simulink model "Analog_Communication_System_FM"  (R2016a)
settings: Solver=ode3  StartTime=0.0  StopTime=6  FixedStep=1/5000000  RelTol=1e-3
libraries: dsparch4 x12, commsynccomp2 x8, simulink x8, commchan3 x2

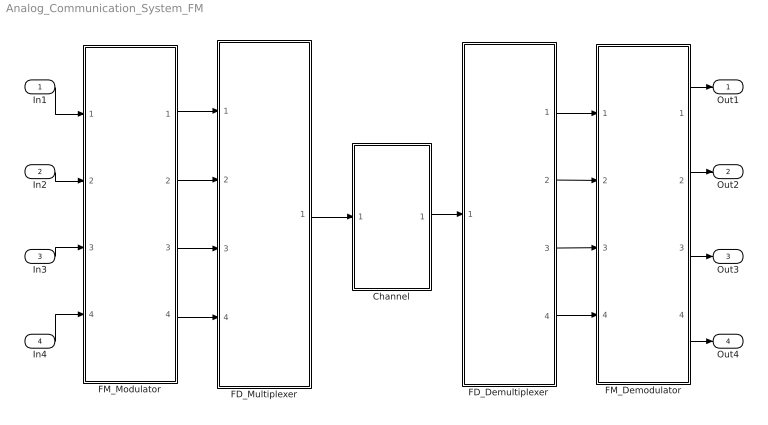
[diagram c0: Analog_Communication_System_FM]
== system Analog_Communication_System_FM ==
  In1 : Inport
  In2 : Inport  Port=2
  In3 : Inport  Port=3
  In4 : Inport  Port=4
  Channel : Subsystem
  FD_Demultiplexer : Subsystem
  FD_Multiplexer : Subsystem
  FM_Demodulator : Subsystem
  FM_Modulator : Subsystem
  Out1 : Outport
  Out2 : Outport  Port=2
  Out3 : Outport  Port=3
  Out4 : Outport  Port=4
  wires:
  In1/1 -> FM_Modulator/1(In1)
  In2/1 -> FM_Modulator/2(In2)
  In3/1 -> FM_Modulator/3(In3)
  In4/1 -> FM_Modulator/4(In4)
  FM_Modulator/1(Out1) -> FD_Multiplexer/1(In1)
  FM_Modulator/2(Out2) -> FD_Multiplexer/2(In2)
  FM_Modulator/3(Out3) -> FD_Multiplexer/3(In3)
  FM_Modulator/4(Out4) -> FD_Multiplexer/4(In4)
  FD_Multiplexer/1(Out) -> Channel/1(In1)
  Channel/1(Out1) -> FD_Demultiplexer/1(Input)
  FD_Demultiplexer/1(Out1) -> FM_Demodulator/1(In1)
  FD_Demultiplexer/2(Out2) -> FM_Demodulator/2(In2)
  FD_Demultiplexer/3(Out3) -> FM_Demodulator/3(In3)
  FD_Demultiplexer/4(Out4) -> FM_Demodulator/4(In4)
  FM_Demodulator/1(Out1) -> Out1/1
  FM_Demodulator/2(Out2) -> Out2/1
  FM_Demodulator/3(Out3) -> Out3/1
  FM_Demodulator/4(Out4) -> Out4/1

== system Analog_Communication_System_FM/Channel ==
  In1 : Inport
  AWGN Channel : commchan3/AWGN Channel  InputProcessing=Columns as channels (frame based)  seed=67  noiseMode="Signal to noise ratio  (Eb/No)"  EbNodB=10  EsNodB=10  SNRdB=10  bitsPerSym=2  Ps=1  Tsym=1/5000000  variance=1
  Releigh Channel : Subsystem
  Reshape1 : Reshape
  Out1 : Outport
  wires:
  In1/1 -> Releigh Channel/1(In1)
  Releigh Channel/1(Out1) -> AWGN Channel/1
  AWGN Channel/1 -> Reshape1/1
  Reshape1/1 -> Out1/1

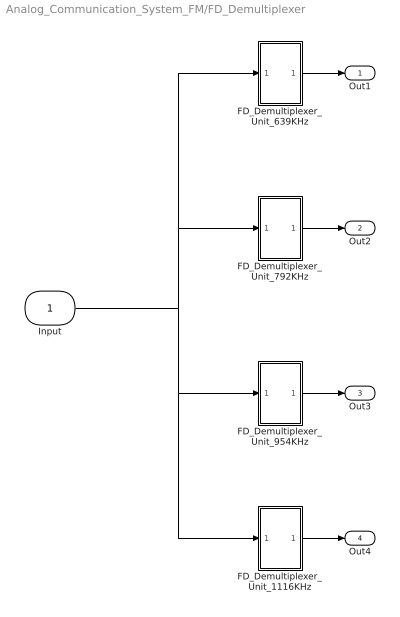
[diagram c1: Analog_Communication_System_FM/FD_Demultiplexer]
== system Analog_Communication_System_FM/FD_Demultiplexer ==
  Input : Inport
  FD_Demultiplexer_Unit_1116KHz : Subsystem
  FD_Demultiplexer_Unit_639KHz : Subsystem
  FD_Demultiplexer_Unit_792KHz : Subsystem
  FD_Demultiplexer_Unit_954KHz : Subsystem
  Out1 : Outport
  Out2 : Outport  Port=2
  Out3 : Outport  Port=3
  Out4 : Outport  Port=4
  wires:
  Input/1 -> FD_Demultiplexer_Unit_1116KHz/1(In1), FD_Demultiplexer_Unit_954KHz/1(In1), FD_Demultiplexer_Unit_792KHz/1(In1), FD_Demultiplexer_Unit_639KHz/1(In1)
  FD_Demultiplexer_Unit_639KHz/1(Out1) -> Out1/1
  FD_Demultiplexer_Unit_792KHz/1(Out1) -> Out2/1
  FD_Demultiplexer_Unit_954KHz/1(Out1) -> Out3/1
  FD_Demultiplexer_Unit_1116KHz/1(Out1) -> Out4/1

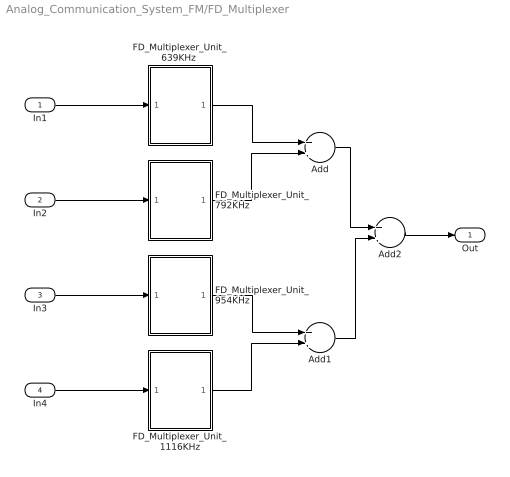
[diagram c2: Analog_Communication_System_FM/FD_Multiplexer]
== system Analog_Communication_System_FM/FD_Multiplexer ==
  In1 : Inport
  In2 : Inport  Port=2
  In3 : Inport  Port=3
  In4 : Inport  Port=4
  Add : Sum
  Add1 : Sum
  Add2 : Sum
  FD_Multiplexer_Unit_1116KHz : Subsystem
  "FD_Multiplexer_Unit_639KHz " : Subsystem
  FD_Multiplexer_Unit_792KHz : Subsystem
  FD_Multiplexer_Unit_954KHz : Subsystem
  Out : Outport
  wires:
  FD_Multiplexer_Unit_792KHz/1(Output) -> Add/2
  "FD_Multiplexer_Unit_639KHz "/1(Output) -> Add/1
  Add/1 -> Add2/1
  Add2/1 -> Out/1
  In2/1 -> FD_Multiplexer_Unit_792KHz/1(Input)
  In1/1 -> "FD_Multiplexer_Unit_639KHz "/1(Input)
  FD_Multiplexer_Unit_954KHz/1(Output) -> Add1/1
  FD_Multiplexer_Unit_1116KHz/1(Output) -> Add1/2
  In3/1 -> FD_Multiplexer_Unit_954KHz/1(Input)
  In4/1 -> FD_Multiplexer_Unit_1116KHz/1(Input)
  Add1/1 -> Add2/2

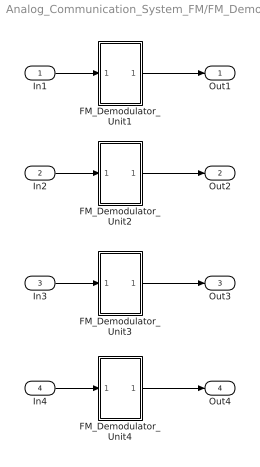
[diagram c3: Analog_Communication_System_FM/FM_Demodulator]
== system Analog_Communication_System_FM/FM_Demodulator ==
  In1 : Inport
  In2 : Inport  Port=2
  In3 : Inport  Port=3
  In4 : Inport  Port=4
  FM_Demodulator_Unit1 : Subsystem
  FM_Demodulator_Unit2 : Subsystem
  FM_Demodulator_Unit3 : Subsystem
  FM_Demodulator_Unit4 : Subsystem
  Out1 : Outport
  Out2 : Outport  Port=2
  Out3 : Outport  Port=3
  Out4 : Outport  Port=4
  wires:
  FM_Demodulator_Unit3/1(Out1) -> Out3/1
  FM_Demodulator_Unit2/1(Out1) -> Out2/1
  FM_Demodulator_Unit4/1(Out1) -> Out4/1
  In1/1 -> FM_Demodulator_Unit1/1(In1)
  In4/1 -> FM_Demodulator_Unit4/1(In1)
  FM_Demodulator_Unit1/1(Out1) -> Out1/1
  In2/1 -> FM_Demodulator_Unit2/1(In1)
  In3/1 -> FM_Demodulator_Unit3/1(In1)

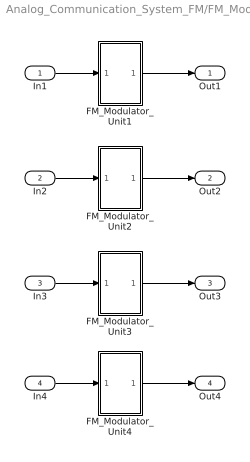
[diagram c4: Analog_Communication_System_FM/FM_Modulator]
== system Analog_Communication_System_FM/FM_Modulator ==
  In1 : Inport
  In2 : Inport  Port=2
  In3 : Inport  Port=3
  In4 : Inport  Port=4
  FM_Modulator_Unit1 : Subsystem
  FM_Modulator_Unit2 : Subsystem
  FM_Modulator_Unit3 : Subsystem
  FM_Modulator_Unit4 : Subsystem
  Out1 : Outport
  Out2 : Outport  Port=2
  Out3 : Outport  Port=3
  Out4 : Outport  Port=4
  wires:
  In1/1 -> FM_Modulator_Unit1/1(In1)
  FM_Modulator_Unit1/1(Out1) -> Out1/1
  In2/1 -> FM_Modulator_Unit2/1(In1)
  FM_Modulator_Unit2/1(Out1) -> Out2/1
  In3/1 -> FM_Modulator_Unit3/1(In1)
  FM_Modulator_Unit3/1(Out1) -> Out3/1
  In4/1 -> FM_Modulator_Unit4/1(In1)
  FM_Modulator_Unit4/1(Out1) -> Out4/1

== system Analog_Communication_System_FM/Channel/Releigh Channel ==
  In1 : Inport
  Complex to Real-Imag : ComplexToRealImag
  Constant1 : Constant  Value=0  SampleTime=1/5000000
  Multipath Rayleigh Fading Channel : commchan3/Multipath Rayleigh Fading Channel  maxDopplerShift=1  spectrumType=Jakes  sigmaGaussian=1/sqrt(2)  coeffRounded=[1 -1.72 0.785]  freqMinMaxRJakes=[0 1]  freqMinMaxAJakes=[0 1]  sigmaGaussian1=1/sqrt(2)  sigmaGaussian2=1/sqrt(2)  centerFreqGaussian1=0.0  centerFreqGaussian2=0.0  gainGaussian1=0.5  gainGaussian2=0.5  coeffBell=9  dopplerSpectrum=doppler.jakes  pathDelays=0  avgPathGaindB=-3  normalizePathGains=on  seed=73  enableProbe=0  openVisAtStart=off  outPathGains=off  outDelay=off
  Real-Imag to Complex : RealImagToComplex
  Out1 : Outport
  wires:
  Real-Imag to Complex/1 -> Multipath Rayleigh Fading Channel/1
  Multipath Rayleigh Fading Channel/1 -> Complex to Real-Imag/1
  Constant1/1 -> Real-Imag to Complex/2
  Complex to Real-Imag/1 -> Out1/1
  Complex to Real-Imag/2 -> ?
  In1/1 -> Real-Imag to Complex/1

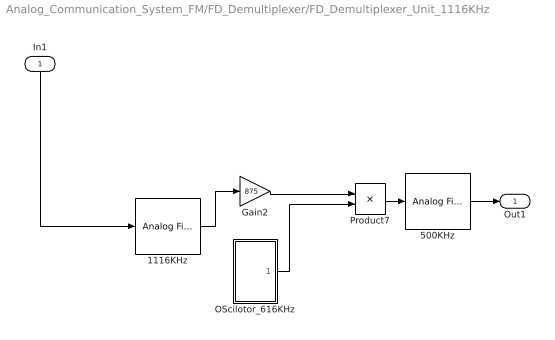
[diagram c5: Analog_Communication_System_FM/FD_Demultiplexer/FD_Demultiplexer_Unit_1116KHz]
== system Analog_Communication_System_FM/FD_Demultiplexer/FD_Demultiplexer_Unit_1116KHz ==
  In1 : Inport
  1116KHz : dsparch4/Analog Filter Design  method=Butterworth  filttype=Bandpass  N=8  Wlo=1066000*2*pi  Whi=1166000*2*pi  Rp=2  Rs=60
  500KHz : dsparch4/Analog Filter Design  method=Butterworth  filttype=Bandpass  N=8  Wlo=450000*2*pi  Whi=550000*2*pi  Rp=2  Rs=40
  Gain2 : Gain  Gain=875
  OScilotor_616KHz : Subsystem
  Product7 : Product
  Out1 : Outport
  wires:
  1116KHz/1 -> Gain2/1
  Gain2/1 -> Product7/1
  OScilotor_616KHz/1(Output) -> Product7/2
  In1/1 -> 1116KHz/1
  Product7/1 -> 500KHz/1
  500KHz/1 -> Out1/1

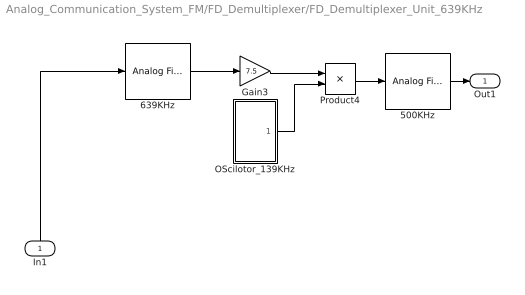
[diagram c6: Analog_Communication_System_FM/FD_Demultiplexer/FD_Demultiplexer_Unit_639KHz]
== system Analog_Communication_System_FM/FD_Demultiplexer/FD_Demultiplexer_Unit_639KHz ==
  In1 : Inport
  500KHz : dsparch4/Analog Filter Design  method=Butterworth  filttype=Bandpass  N=8  Wlo=450000*2*pi  Whi=550000*2*pi  Rp=2  Rs=40
  639KHz : dsparch4/Analog Filter Design  method=Butterworth  filttype=Bandpass  N=8  Wlo=589000*2*pi  Whi=689000*2*pi  Rp=2  Rs=40
  Gain3 : Gain  Gain=7.5
  OScilotor_139KHz : Subsystem
  Product4 : Product
  Out1 : Outport
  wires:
  639KHz/1 -> Gain3/1
  OScilotor_139KHz/1(Output) -> Product4/2
  Gain3/1 -> Product4/1
  In1/1 -> 639KHz/1
  500KHz/1 -> Out1/1
  Product4/1 -> 500KHz/1

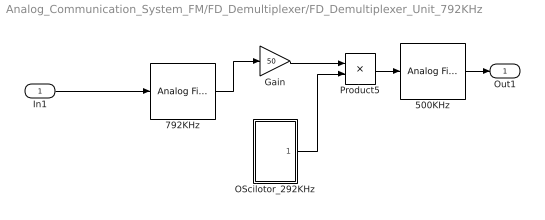
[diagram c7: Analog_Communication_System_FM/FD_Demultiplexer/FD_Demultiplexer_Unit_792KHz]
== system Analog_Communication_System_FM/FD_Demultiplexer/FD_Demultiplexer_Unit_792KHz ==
  In1 : Inport
  500KHz : dsparch4/Analog Filter Design  method=Butterworth  filttype=Bandpass  N=8  Wlo=450000*2*pi  Whi=550000*2*pi  Rp=2  Rs=40
  792KHz : dsparch4/Analog Filter Design  method=Butterworth  filttype=Bandpass  N=8  Wlo=742000*2*pi  Whi=842000*2*pi  Rp=2  Rs=40
  Gain : Gain  Gain=50
  OScilotor_292KHz : Subsystem
  Product5 : Product
  Out1 : Outport
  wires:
  Gain/1 -> Product5/1
  792KHz/1 -> Gain/1
  OScilotor_292KHz/1(Output) -> Product5/2
  In1/1 -> 792KHz/1
  Product5/1 -> 500KHz/1
  500KHz/1 -> Out1/1

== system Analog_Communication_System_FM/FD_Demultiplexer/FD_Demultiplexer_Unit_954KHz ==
  In1 : Inport
  500KHz : dsparch4/Analog Filter Design  method=Butterworth  filttype=Bandpass  N=8  Wlo=450000*2*pi  Whi=550000*2*pi  Rp=2  Rs=40
  954KHz : dsparch4/Analog Filter Design  method=Butterworth  filttype=Bandpass  N=8  Wlo=904000*2*pi  Whi=1004000*2*pi  Rp=2  Rs=40
  Gain1 : Gain  Gain=100
  OScilotor_454KHz : Subsystem
  Product6 : Product
  Out1 : Outport
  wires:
  OScilotor_454KHz/1(Output) -> Product6/2
  954KHz/1 -> Gain1/1
  Gain1/1 -> Product6/1
  In1/1 -> 954KHz/1
  Product6/1 -> 500KHz/1
  500KHz/1 -> Out1/1

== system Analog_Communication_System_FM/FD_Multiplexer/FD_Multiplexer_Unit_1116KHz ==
  Input : Inport
  Carrier Generator : Subsystem
  Product : Product
  Output : Outport
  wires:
  Input/1 -> Product/1
  Product/1 -> Output/1
  Carrier Generator/1(Carrier) -> Product/2

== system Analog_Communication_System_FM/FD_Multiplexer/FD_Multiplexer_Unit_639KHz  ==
  Input : Inport
  Carrier Generator : Subsystem
  Product : Product
  Output : Outport
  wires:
  Product/1 -> Output/1
  Input/1 -> Product/1
  Carrier Generator/1(Carrier) -> Product/2

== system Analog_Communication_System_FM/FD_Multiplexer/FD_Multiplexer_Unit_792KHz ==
  Input : Inport
  Carrier Generator : Subsystem
  Product : Product
  Output : Outport
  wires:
  Product/1 -> Output/1
  Input/1 -> Product/1
  Carrier Generator/1(Carrier) -> Product/2

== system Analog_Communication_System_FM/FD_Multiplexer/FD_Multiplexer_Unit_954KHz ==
  Input : Inport
  Carrier Generator : Subsystem
  Product : Product
  Output : Outport
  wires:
  Input/1 -> Product/1
  Product/1 -> Output/1
  Carrier Generator/1(Carrier) -> Product/2

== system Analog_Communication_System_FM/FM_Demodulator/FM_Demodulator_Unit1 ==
  In1 : Inport
  Analog Filter Design : dsparch4/Analog Filter Design  method=Butterworth  filttype=Lowpass  N=10  Wlo=45000*2*pi  Whi=80  Rp=2  Rs=40
  Derivative : Derivative
  Product1 : Product
  Sine Wave1 : Sin  Frequency=500000*2*pi  Phase=-1.5*pi
  Out1 : Outport
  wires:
  Analog Filter Design/1 -> Out1/1
  Product1/1 -> Derivative/1
  Sine Wave1/1 -> Product1/2
  In1/1 -> Product1/1
  Derivative/1 -> Analog Filter Design/1

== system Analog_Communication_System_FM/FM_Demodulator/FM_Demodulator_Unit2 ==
  In1 : Inport
  Analog Filter Design : dsparch4/Analog Filter Design  method=Butterworth  filttype=Lowpass  N=10  Wlo=45000*2*pi  Whi=80  Rp=2  Rs=40
  Derivative : Derivative
  Product1 : Product
  Sine Wave1 : Sin  Frequency=500000*2*pi  Phase=-1.5*pi
  Out1 : Outport
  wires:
  Analog Filter Design/1 -> Out1/1
  Product1/1 -> Derivative/1
  Sine Wave1/1 -> Product1/2
  In1/1 -> Product1/1
  Derivative/1 -> Analog Filter Design/1

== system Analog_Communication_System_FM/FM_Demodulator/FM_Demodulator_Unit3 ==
  In1 : Inport
  Analog Filter Design : dsparch4/Analog Filter Design  method=Butterworth  filttype=Lowpass  N=10  Wlo=45000*2*pi  Whi=80  Rp=2  Rs=40
  Derivative : Derivative
  Product1 : Product
  Sine Wave1 : Sin  Frequency=500000*2*pi  Phase=-1.5*pi
  Out1 : Outport
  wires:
  Analog Filter Design/1 -> Out1/1
  Product1/1 -> Derivative/1
  Sine Wave1/1 -> Product1/2
  In1/1 -> Product1/1
  Derivative/1 -> Analog Filter Design/1

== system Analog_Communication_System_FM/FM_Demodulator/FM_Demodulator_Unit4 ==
  In1 : Inport
  Analog Filter Design : dsparch4/Analog Filter Design  method=Butterworth  filttype=Lowpass  N=10  Wlo=45000*2*pi  Whi=80  Rp=2  Rs=40
  Derivative : Derivative
  Product1 : Product
  Sine Wave1 : Sin  Frequency=500000*2*pi  Phase=-1.5*pi
  Out1 : Outport
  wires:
  Analog Filter Design/1 -> Out1/1
  Product1/1 -> Derivative/1
  Sine Wave1/1 -> Product1/2
  In1/1 -> Product1/1
  Derivative/1 -> Analog Filter Design/1

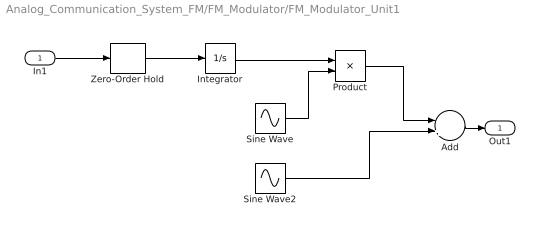
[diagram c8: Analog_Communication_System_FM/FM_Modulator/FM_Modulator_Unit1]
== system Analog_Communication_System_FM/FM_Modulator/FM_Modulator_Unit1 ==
  In1 : Inport
  Add : Sum  Inputs=-+
  Integrator : Integrator
  Product : Product
  Sine Wave : Sin  Frequency=500000*2*pi  Phase=-0.5*pi
  Sine Wave2 : Sin  Frequency=500000*2*pi
  Zero-Order Hold : ZeroOrderHold  SampleTime=1/5000000
  Out1 : Outport
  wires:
  Zero-Order Hold/1 -> Integrator/1
  In1/1 -> Zero-Order Hold/1
  Sine Wave/1 -> Product/2
  Sine Wave2/1 -> Add/2
  Product/1 -> Add/1
  Integrator/1 -> Product/1
  Add/1 -> Out1/1

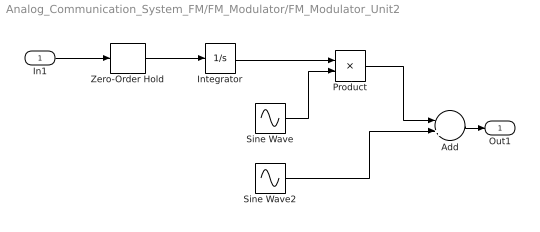
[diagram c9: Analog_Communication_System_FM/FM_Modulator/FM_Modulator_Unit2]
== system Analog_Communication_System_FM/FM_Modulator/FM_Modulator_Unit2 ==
  In1 : Inport
  Add : Sum  Inputs=-+
  Integrator : Integrator
  Product : Product
  Sine Wave : Sin  Frequency=500000*2*pi  Phase=-0.5*pi
  Sine Wave2 : Sin  Frequency=500000*2*pi
  Zero-Order Hold : ZeroOrderHold  SampleTime=1/5000000
  Out1 : Outport
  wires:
  Zero-Order Hold/1 -> Integrator/1
  In1/1 -> Zero-Order Hold/1
  Sine Wave/1 -> Product/2
  Sine Wave2/1 -> Add/2
  Product/1 -> Add/1
  Integrator/1 -> Product/1
  Add/1 -> Out1/1

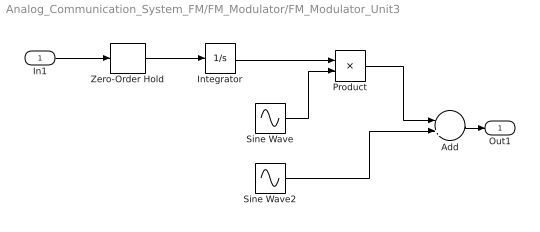
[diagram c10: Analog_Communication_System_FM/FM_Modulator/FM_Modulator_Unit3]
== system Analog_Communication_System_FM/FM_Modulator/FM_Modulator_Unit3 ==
  In1 : Inport
  Add : Sum  Inputs=-+
  Integrator : Integrator
  Product : Product
  Sine Wave : Sin  Frequency=500000*2*pi  Phase=-0.5*pi
  Sine Wave2 : Sin  Frequency=500000*2*pi
  Zero-Order Hold : ZeroOrderHold  SampleTime=1/5000000
  Out1 : Outport
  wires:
  Zero-Order Hold/1 -> Integrator/1
  In1/1 -> Zero-Order Hold/1
  Sine Wave/1 -> Product/2
  Sine Wave2/1 -> Add/2
  Product/1 -> Add/1
  Integrator/1 -> Product/1
  Add/1 -> Out1/1

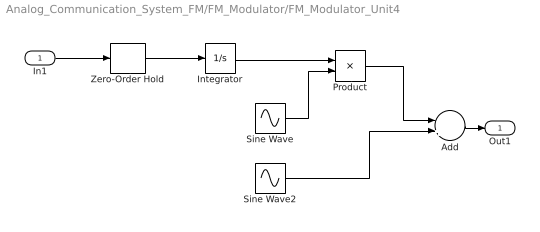
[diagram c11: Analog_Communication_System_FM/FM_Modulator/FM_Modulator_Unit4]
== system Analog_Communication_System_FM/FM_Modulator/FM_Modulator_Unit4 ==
  In1 : Inport
  Add : Sum  Inputs=-+
  Integrator : Integrator
  Product : Product
  Sine Wave : Sin  Frequency=500000*2*pi  Phase=-0.5*pi
  Sine Wave2 : Sin  Frequency=500000*2*pi
  Zero-Order Hold : ZeroOrderHold  SampleTime=1/5000000
  Out1 : Outport
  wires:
  Zero-Order Hold/1 -> Integrator/1
  In1/1 -> Zero-Order Hold/1
  Sine Wave/1 -> Product/2
  Sine Wave2/1 -> Add/2
  Product/1 -> Add/1
  Integrator/1 -> Product/1
  Add/1 -> Out1/1

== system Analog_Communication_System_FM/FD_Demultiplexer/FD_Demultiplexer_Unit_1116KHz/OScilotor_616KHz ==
  Constant : Constant
  Discrete-Time VCO : commsynccomp2/Discrete-Time VCO  Ac=1  Fc=0  Kc=1000  Ph=0  ts=1/5000000
  Slider Gain : simulink/Math Operations/Slider Gain  low=616  gain=616  high=2070
  Output : Outport
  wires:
  Constant/1 -> Slider Gain/1
  Slider Gain/1 -> Discrete-Time VCO/1
  Discrete-Time VCO/1 -> Output/1

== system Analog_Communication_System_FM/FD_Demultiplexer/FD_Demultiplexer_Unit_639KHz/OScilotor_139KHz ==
  Constant : Constant
  Discrete-Time VCO : commsynccomp2/Discrete-Time VCO  Ac=1  Fc=0  Kc=1000  Ph=0  ts=1/5000000
  Slider Gain : simulink/Math Operations/Slider Gain  low=139  gain=139  high=2070
  Output : Outport
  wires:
  Constant/1 -> Slider Gain/1
  Slider Gain/1 -> Discrete-Time VCO/1
  Discrete-Time VCO/1 -> Output/1

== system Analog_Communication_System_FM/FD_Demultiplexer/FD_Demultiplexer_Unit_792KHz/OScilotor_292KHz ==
  Constant : Constant
  Discrete-Time VCO : commsynccomp2/Discrete-Time VCO  Ac=1  Fc=0  Kc=1000  Ph=0  ts=1/5000000
  Slider Gain : simulink/Math Operations/Slider Gain  low=292  gain=292  high=2070
  Output : Outport
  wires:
  Constant/1 -> Slider Gain/1
  Slider Gain/1 -> Discrete-Time VCO/1
  Discrete-Time VCO/1 -> Output/1

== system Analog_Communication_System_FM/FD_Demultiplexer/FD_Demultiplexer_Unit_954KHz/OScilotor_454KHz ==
  Constant : Constant
  Discrete-Time VCO : commsynccomp2/Discrete-Time VCO  Ac=1  Fc=0  Kc=1000  Ph=0  ts=1/5000000
  Slider Gain : simulink/Math Operations/Slider Gain  low=454  gain=454  high=2070
  Output : Outport
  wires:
  Constant/1 -> Slider Gain/1
  Slider Gain/1 -> Discrete-Time VCO/1
  Discrete-Time VCO/1 -> Output/1

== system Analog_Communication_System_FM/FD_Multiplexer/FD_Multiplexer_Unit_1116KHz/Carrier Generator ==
  Constant1 : Constant
  Discrete-Time VCO : commsynccomp2/Discrete-Time VCO  Ac=1  Fc=0  Kc=1000  Ph=0  ts=1/5000000
  Slider Gain : simulink/Math Operations/Slider Gain  low=550  gain=616  high=2500
  Carrier : Outport
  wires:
  Discrete-Time VCO/1 -> Carrier/1
  Slider Gain/1 -> Discrete-Time VCO/1
  Constant1/1 -> Slider Gain/1

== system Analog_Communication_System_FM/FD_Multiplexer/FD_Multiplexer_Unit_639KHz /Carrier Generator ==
  Constant1 : Constant
  Discrete-Time VCO : commsynccomp2/Discrete-Time VCO  Ac=1  Fc=0  Kc=1000  Ph=0  ts=1/5000000
  Slider Gain : simulink/Math Operations/Slider Gain  low=0  gain=139  high=1605
  Carrier : Outport
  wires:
  Discrete-Time VCO/1 -> Carrier/1
  Slider Gain/1 -> Discrete-Time VCO/1
  Constant1/1 -> Slider Gain/1

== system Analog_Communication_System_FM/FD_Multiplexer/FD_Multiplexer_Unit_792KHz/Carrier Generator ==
  Constant1 : Constant
  Discrete-Time VCO : commsynccomp2/Discrete-Time VCO  Ac=1  Fc=0  Kc=1000  Ph=0  ts=1/5000000
  Slider Gain : simulink/Math Operations/Slider Gain  low=292  gain=292  high=1605
  Carrier : Outport
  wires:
  Discrete-Time VCO/1 -> Carrier/1
  Slider Gain/1 -> Discrete-Time VCO/1
  Constant1/1 -> Slider Gain/1

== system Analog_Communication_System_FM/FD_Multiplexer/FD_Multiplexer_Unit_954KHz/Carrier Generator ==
  Constant1 : Constant
  Discrete-Time VCO : commsynccomp2/Discrete-Time VCO  Ac=1  Fc=0  Kc=1000  Ph=0  ts=1/5000000
  Slider Gain : simulink/Math Operations/Slider Gain  low=454  gain=454  high=1605
  Carrier : Outport
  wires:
  Discrete-Time VCO/1 -> Carrier/1
  Slider Gain/1 -> Discrete-Time VCO/1
  Constant1/1 -> Slider Gain/1
